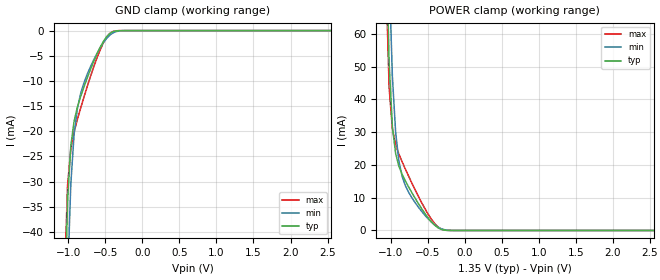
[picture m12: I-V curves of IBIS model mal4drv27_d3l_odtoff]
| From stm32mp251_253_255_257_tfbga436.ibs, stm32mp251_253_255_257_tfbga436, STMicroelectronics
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[Model] mal4drv27_d3l_odtoff
Model_type   Input
Polarity   Non-Inverting
Enable   Active-High
C_comp   1.684pF   1.663pF   1.711pF
C_comp_pullup   812.334fF   800.254fF   826.800fF
C_comp_pulldown   769.309fF   756.111fF   787.425fF
Vinh = 805.000mV
Vinl = 545.000mV
[Model Spec]
D_overshoot_ampl_h 0.4 NA   NA
D_overshoot_ampl_l 0.4 NA   NA
D_overshoot_area_l 110.000m NA   NA
D_overshoot_area_h 110.000m NA   NA
[Temperature Range]   25.000   125.000   -40.000
[Voltage Range]   1.350V   1.283V   1.425V
[GND Clamp Reference]   0.00V   0.00V   0.00V
[C Comp Corner]
| variable   typ   min   max
C_comp   1.684pF   1.663pF   1.711pF
C_comp_pullup   812.334fF   800.254fF   826.800fF
C_comp_pulldown   769.309fF   756.111fF   787.425fF
[POWER Clamp Reference]   1.350V   1.283V   1.425V
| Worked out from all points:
|   GND clamp passes 1 mA (typ) near -0.47 V on its own axis
|   POWER clamp passes 1 mA (typ) near -0.37 V on its own axis
[GND Clamp]
-1.318V   -672mA     -638mA     -661.1mA
-1.054V   -60.41mA   -84.99mA   -50.75mA
-1.011V   -34.02mA   -49.92mA   -30.84mA
-966.7mV  -22.91mA   -30.54mA   -23.58mA
-922.7mV  -18.04mA   -20.68mA   -20.16mA
-878.8mV  -15.25mA   -15.56mA   -17.69mA
-834.8mV  -13.14mA   -12.55mA   -15.44mA
-747mV    -9.486mA   -8.743mA   -11.21mA
-615.2mV  -4.709mA   -4.591mA   -5.504mA
-439.4mV  -562.2uA   -889.5uA   -546.1uA
-219.7mV  -954.1nA   -9.356uA   -215nA
2.68V     18.98nA    945nA      23.53nA
[Power Clamp]
-1.33V    889mA      842.2mA    872.8mA
-1.067V   94.44mA    130.9mA    77.96mA
-1.023V   51.04mA    78.45mA    43.53mA
-978.8mV  31.54mA    46.94mA    31.01mA
-934.8mV  23.45mA    29.85mA    26.15mA
-890.9mV  19.58mA    21.13mA    23.3mA
-847mV    17.11mA    16.47mA    20.93mA
-671.2mV  9.815mA    8.474mA    12.37mA
-495.5mV  3.823mA    3.529mA    4.955mA
-363.6mV  819.5uA    1.024mA    1.072mA
-187.9mV  4.227uA    28.6uA     2.566uA
2.668V    -29.12nA   -796.8nA   -15.73nA
